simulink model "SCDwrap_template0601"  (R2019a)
settings: configuration reference "configurationSettings" (kept in a data dictionary, not in this file)
undefined symbols (not defined in the file or in its folder): SCDnode06params

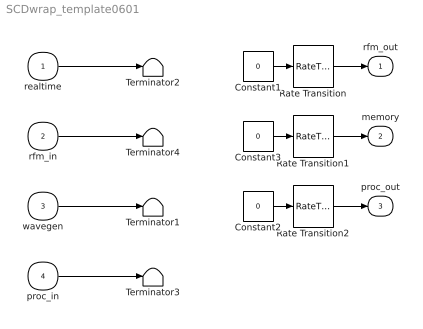
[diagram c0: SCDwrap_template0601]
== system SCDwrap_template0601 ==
  realtime : Inport  OutDataTypeStr=single  SampleTime=SCDnode06params.timing.thperiod(1)
  rfm_in : Inport  Port=2  OutDataTypeStr=Bus: RFMINbus  SampleTime=SCDnode06params.timing.thperiod(1)
  wavegen : Inport  Port=3  OutDataTypeStr=Bus: WG0601bus  SampleTime=SCDnode06params.timing.thperiod(1)
  proc_in : Inport  Port=4  OutDataTypeStr=Bus: PROCIN06bus  SampleTime=SCDnode06params.timing.thperiod(1)
  Constant1 : Constant  Value=0  OutDataTypeStr=Bus: RFMOUT06bus
  Constant2 : Constant  Value=0  OutDataTypeStr=Bus: PROCOUT0601bus
  Constant3 : Constant  Value=0  OutDataTypeStr=Bus: MEM0601bus
  Rate Transition : RateTransition
  Rate Transition1 : RateTransition
  Rate Transition2 : RateTransition
  Terminator{1..4} (4 alike) : Terminator
  rfm_out : Outport  OutDataTypeStr=Bus: RFMOUT06bus  SampleTime=SCDnode06params.timing.thperiod(1)
  memory : Outport  Port=2  OutDataTypeStr=Bus: MEM0601bus  SampleTime=SCDnode06params.timing.thperiod(1)
  proc_out : Outport  Port=3  OutDataTypeStr=Bus: PROCOUT0601bus  SampleTime=SCDnode06params.timing.thperiod(1)
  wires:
  Constant1/1 -> Rate Transition/1
  Constant2/1 -> Rate Transition2/1
  Constant3/1 -> Rate Transition1/1
  rfm_in/1 -> Terminator4/1
  wavegen/1 -> Terminator1/1
  proc_in/1 -> Terminator3/1
  Rate Transition/1 -> rfm_out/1
  Rate Transition1/1 -> memory/1
  Rate Transition2/1 -> proc_out/1
  realtime/1 -> Terminator2/1
